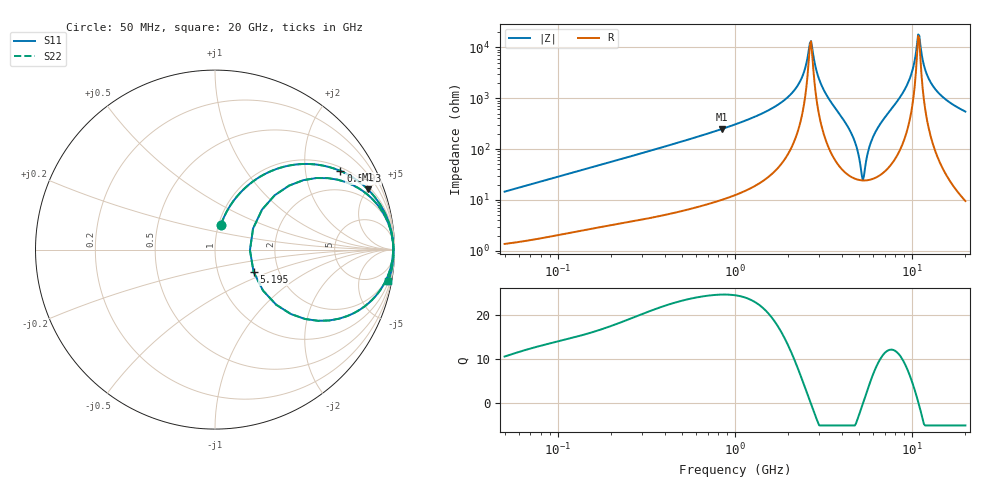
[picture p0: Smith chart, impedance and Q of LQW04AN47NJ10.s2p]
!Murata Part Number: LQW04AN47NJ10
!These Parameters are Measured in Series Mode Connection
!  o--[Z]--o
!Port1  Port2
!  o-------o
!Freq. Start=50[MHz] Stop=20[GHz], 401[Steps]
# Hz S RI R 50
!Freq.(Hz) S11(Real) S11(Imag) S21(Real) S21(Imag) S12(Real) S12(Imag) S22(Real) S22(Imag)
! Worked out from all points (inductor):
!   401 points, 50 MHz to 20 GHz, reference 50 ohm
!   read as one part in series: L = 45.9 nH near 51.52 MHz
!   highest Q = 24.7 at 848.1 MHz (marker M1), where L = 46.8 nH
!   self-resonance near 2.647 GHz
!   S11 on the Smith chart (normalised r, x): 50 MHz: 1.03, +0.29; 549.3 MHz: 1.13, +3.10; 5.195 GHz: 1.49, -0.39; 20 GHz: 1, -11
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5e7  0.0333 0.1383  0.9667 -0.1383  0.9667 -0.1383  0.0333 0.1383
1.364002e8  0.1457 0.3219  0.8543 -0.3219  0.8543 -0.3219  0.1457 0.3219
3.721004e8  0.5185 0.4771  0.4815 -0.4771  0.4815 -0.4771  0.5185 0.4771
5.492803e8  0.6987 0.4382  0.3013 -0.4382  0.3013 -0.4382  0.6987 0.4382
8.480927e8  0.8521 0.3353  0.1479 -0.3353  0.1479 -0.3353  0.8521 0.3353
1e9  0.8932 0.2891  0.1068 -0.2891  0.1068 -0.2891  0.8932 0.2891
2.021818e9  0.9851 0.088  0.0149 -0.088  0.0149 -0.088  0.9851 0.088
2.348516e9  0.9912 0.043  0.00878 -0.043  0.00878 -0.043  0.9912 0.043
2.647493e9  0.9927 0.00386  0.00728 -0.00386  0.00728 -0.00386  0.9927 0.00386
2.728004e9  0.9925 -0.00664  0.00749 0.00664  0.00749 0.00664  0.9925 -0.00664
3.121702e9  0.9874 -0.0596  0.0126 0.0596  0.0126 0.0596  0.9874 -0.0596
4.275624e9  0.8746 -0.2808  0.1254 0.2808  0.1254 0.2808  0.8746 -0.2808
4.81993e9  0.5751 -0.3968  0.4249 0.3968  0.4249 0.3968  0.5751 -0.3968
5.194772e9  0.2149 -0.124  0.7851 0.124  0.7851 0.124  0.2149 -0.124
5.769027e9  0.5649 0.3988  0.4351 -0.3988  0.4351 -0.3988  0.5649 0.3988
6.406762e9  0.8482 0.3078  0.1518 -0.3078  0.1518 -0.3078  0.8482 0.3078
7.442007e9  0.9544 0.1713  0.0456 -0.1713  0.0456 -0.1713  0.9544 0.1713
9.457416e9  0.9908 0.0497  0.0092 -0.0497  0.0092 -0.0497  0.9908 0.0497
1.082228e10  0.9948 0.00191  0.00522 -0.00191  0.00522 -0.00191  0.9948 0.00191
1.201863e10  0.9945 -0.031  0.00548 0.031  0.00548 0.031  0.9945 -0.031
1.314879e10  0.9926 -0.0575  0.00744 0.0575  0.00744 0.0575  0.9926 -0.0575
2e10  0.9647 -0.1759  0.0353 0.1759  0.0353 0.1759  0.9647 -0.1759
